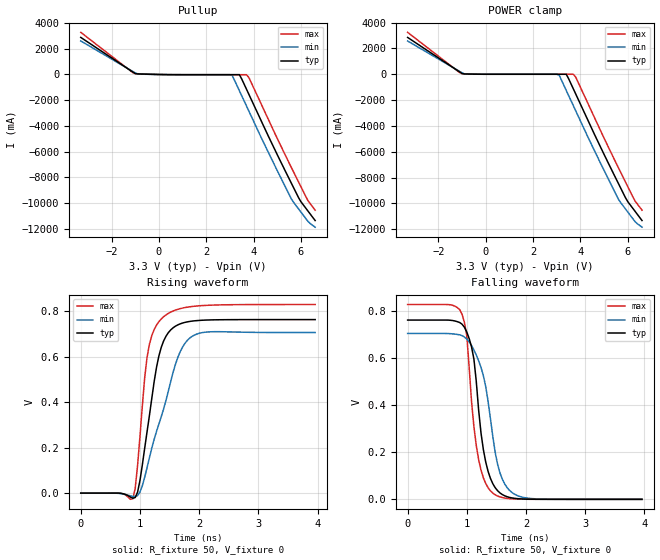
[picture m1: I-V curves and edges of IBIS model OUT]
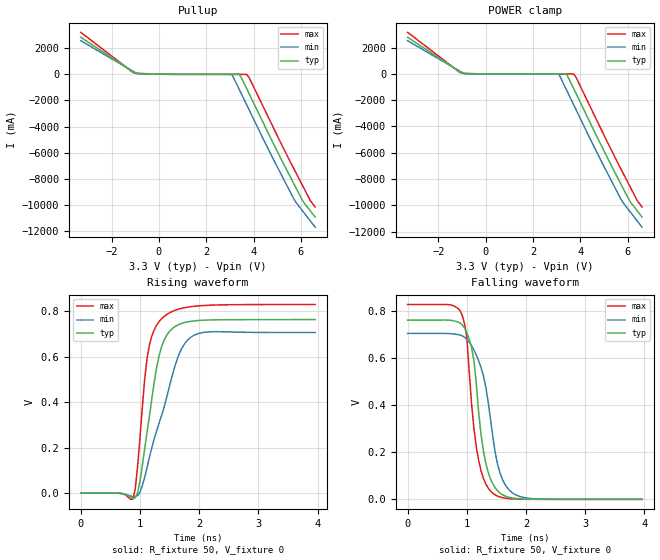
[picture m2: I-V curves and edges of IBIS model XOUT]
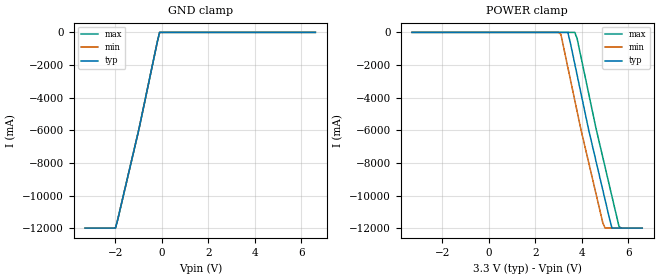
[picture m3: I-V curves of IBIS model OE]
|   IBIS File sg3225hbn_33v.ibs
[IBIS Ver]   3.2
[File name]   sg3225hbn_33v.ibs
[File Rev]   1.0
[Date]   April 7, 2016
[Source]
[Disclaimer]
Seiko Epson Corporation makes no warranty with respect to the information
contained herein.
[Copyright]
Copyright(C) 2013, Seiko Epson Corporation. All rights reserved.
|   Component SG3225HBN 3.3V
[Component]   sg3225hbn_33v
[Manufacturer]   Seiko Epson Corporation
[Package]
R_pkg   0.048   NA   NA
L_pkg   0.48n   NA   NA
C_pkg   0.21p   NA   NA
[Pin] signal_name   model_name   R_pin   L_pin   C_pin
1   OE   OE
2   NC   NC
3   GND   GND
4   OUT   OUT   0.048   0.48n   0.21p
5   XOUT   XOUT   0.048   0.48n   0.21p
6   VCC   POWER
[Diff Pin] inv_pin vdiff   tdelay_typ
4   5   0   0
| Models and submodels in the file (3): OUT (Open_source), XOUT (Open_source), OE (Input)
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[Model]   OUT
Model_type Open_source
Enable Active-High
Polarity Non-Inverting
Vref=0
Vmeas=0.375
Rref=50
Cref=0
C_comp   3.20p   2.99p   3.64p
[Temperature Range] 25   85   -40
[Voltage Range]   3.3   2.97   3.63
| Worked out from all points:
|   slope of the pullup table from 0 to 0.495 V, typ, clamps not added: 39.7 ohm
|   POWER clamp passes 1 mA (typ) near -0.15 V on its own axis
|   falling waveform, R_fixture 50, V_fixture 0: 20-80 % time 216ps typ, 293ps min, 193ps max; typ from 0.763 V to 0 V
|   rising waveform, R_fixture 50, V_fixture 0: 20-80 % time 272ps typ, 451ps min, 195ps max; typ from 0 V to 0.763 V
[Pullup]
-3.3V     2.881A     2.607A     3.275A
-1V       78.43mA    123.5mA    70.06mA
-500mV    22.06mA    15.05mA    31.55mA
3V        -15.31mA   -14.25mA   -16.57mA
3.1V      -15.31mA   -78.05mA   -16.61mA
3.4V      -15.31mA   -1.262A    -16.66mA
3.7V      -1.144A    -2.447A    -16.68mA
3.8V      -1.539A    -2.842A    -236.3mA
5.6V      -8.462A    -9.681A    -7.243A
6V        -9.884A    -10.69A    -8.721A
6.3V      -10.61A    -11.42A    -9.812A
6.6V      -11.34A    -11.86A    -10.54A
[POWER Clamp]
-3.3V     2.853A     2.578A     3.249A
-1V       61.1mA     110.8mA    46.56mA
-700mV    15.18mA    8.186mA    27.06mA
3V        -158.7pA   -183.6pA   -141pA
3.1V      -166.7pA   -69.76mA   -149pA
3.4V      -190.7pA   -1.254A    -173pA
3.7V      -1.136A    -2.439A    -197pA
3.8V      -1.531A    -2.834A    -227.1mA
5.6V      -8.453A    -9.673A    -7.234A
6V        -9.874A    -10.68A    -8.712A
6.3V      -10.6A     -11.41A    -9.801A
6.6V      -11.33A    -11.84A    -10.53A
[Falling Waveform]
R_fixture=50
V_fixture=0
V_fixture_min=0
V_fixture_max=0
0s        763.3mV    706.4mV    829.6mV
920ps     745.7mV    697mV      787.6mV
1ns       712.2mV    682.3mV    696.5mV
1.08ns    649.1mV    654.8mV    415.8mV
1.2ns     379.3mV    589.9mV    169mV
1.32ns    158.2mV    478.9mV    67.16mV
1.44ns    66.19mV    266mV      26.37mV
1.6ns     20.28mV    85.77mV    7.546mV
1.84ns    3.312mV    17.45mV    1.174mV
3.96ns    0V         0V         0V
[Rising Waveform]
R_fixture=50
V_fixture=0
V_fixture_min=0
V_fixture_max=0
0s        0V         1.468uV    0V
880ps     -22.25mV   -14.76mV   -25mV
960ps     4.283mV    -10.74mV   121.6mV
1.08ns    197.1mV    69.39mV    507.5mV
1.12ns    269.5mV    111.9mV    596.9mV
1.28ns    553.2mV    271.5mV    738.8mV
1.4ns     669.2mV    370.3mV    775.8mV
1.68ns    744.4mV    622.1mV    811.3mV
1.92ns    757.7mV    695mV      821.9mV
3.96ns    763.3mV    706.3mV    829.6mV
[Ramp]
R_load=50
dV/dt_r   4.580E-1/2.704E-10   4.238E-1/4.510E-10   4.978E-1/1.934E-10
dV/dt_f   4.580E-1/2.127E-10   4.238E-1/2.913E-10   4.978E-1/1.879E-10
|[End   OUT
[Model]   XOUT
Model_type Open_source
Enable Active-High
Polarity Inverting
Vref=0
Vmeas=0.375
Rref=50
Cref=0
C_comp   3.20p   2.99p   3.64p
[Temperature Range] 25   85   -40
[Voltage Range]   3.3   2.97   3.63
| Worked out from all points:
|   slope of the pullup table from 0 to 0.495 V, typ, clamps not added: 39.7 ohm
|   POWER clamp passes 1 mA (typ) near -0.15 V on its own axis
|   falling waveform, R_fixture 50, V_fixture 0: 20-80 % time 216ps typ, 293ps min, 192ps max; typ from 0.763 V to 0 V
|   rising waveform, R_fixture 50, V_fixture 0: 20-80 % time 273ps typ, 452ps min, 197ps max; typ from 0 V to 0.763 V
[Pullup]
-3.3V     2.816A     2.555A     3.19A
-1V       77.27mA    121mA      69.81mA
-700mV    32.22mA    22.26mA    45.41mA
3.1V      -15.31mA   -73.56mA   -16.61mA
3.4V      -15.31mA   -1.191A    -16.66mA
3.7V      -1.08A     -2.31A     -16.68mA
3.8V      -1.453A    -2.683A    -222.4mA
4.7V      -4.806A    -5.998A    -3.579A
5.7V      -8.368A    -9.524A    -7.213A
6.1V      -9.742A    -10.51A    -8.614A
6.4V      -10.44A    -11.21A    -9.663A
6.6V      -10.91A    -11.68A    -10.14A
[POWER Clamp]
-3.3V     2.789A     2.526A     3.165A
-1V       60.1mA     108.6mA    46.38mA
-800mV    18.78mA    11.85mA    32.09mA
3.1V      -166.7pA   -66.07mA   -149pA
3.4V      -190.7pA   -1.184A    -173pA
3.7V      -1.072A    -2.303A    -197pA
3.8V      -1.445A    -2.676A    -214.5mA
4.7V      -4.798A    -5.991A    -3.571A
5.7V      -8.361A    -9.516A    -7.205A
6.1V      -9.734A    -10.5A     -8.606A
6.4V      -10.43A    -11.2A     -9.654A
6.6V      -10.9A     -11.67A    -10.13A
[Falling Waveform]
R_fixture=50
V_fixture=0
V_fixture_min=0
V_fixture_max=0
0s        763.3mV    706.4mV    829.6mV
920ps     744.3mV    696.5mV    785.5mV
1ns       710.4mV    681.8mV    691mV
1.08ns    646.7mV    654.5mV    406.6mV
1.2ns     370.9mV    590mV      165.3mV
1.32ns    155.2mV    478.7mV    65.67mV
1.44ns    64.98mV    265.6mV    25.78mV
1.6ns     19.89mV    85.9mV     7.377mV
1.84ns    3.241mV    17.51mV    1.149mV
3.96ns    0V         0V         0V
[Rising Waveform]
R_fixture=50
V_fixture=0
V_fixture_min=0
V_fixture_max=0
0s        0V         1.183uV    0V
880ps     -22.39mV   -14.95mV   -26.37mV
960ps     2.08mV     -10.93mV   116.5mV
1.08ns    194.8mV    70.06mV    502mV
1.12ns    267.4mV    112.9mV    592.6mV
1.28ns    549.9mV    272.8mV    737.5mV
1.4ns     667.5mV    371mV      775.1mV
1.68ns    744.1mV    622.2mV    811.1mV
1.92ns    757.6mV    695mV      821.8mV
3.96ns    763.3mV    706.3mV    829.6mV
[Ramp]
R_load=50
dV/dt_r   4.580E-1/2.716E-10   4.238E-1/4.519E-10   4.978E-1/1.946E-10
dV/dt_f   4.580E-1/2.127E-10   4.238E-1/2.912E-10   4.978E-1/1.880E-10
|[End   XOUT
[Model]   OE
Model_type Input
Vinh=2.31
Vinl=0.99
C_comp   3p   3p   3p
[Temperature Range] 25   85   -40
[Voltage Range]   3.3   2.97   3.63
[POWER Clamp Reference]3.3   2.97   3.63
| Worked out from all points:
|   GND clamp passes 1 mA (typ) near -0.10 V on its own axis
[GND Clamp]
-3.3V     -12A       -12A       -12A
-2V       -12A       -12A       -12A
-1.9V     -11.47A    -11.47A    -11.47A
-1V       -6A        -6A        -6A
-200mV    -592.5mA   -592.5mA   -592.5mA
-100mV    -33.15uA   -29.16uA   -40.33uA
6.6V      32.19uA    34.53uA    32.12uA
[POWER Clamp]
-3.3V     32.19uA    31.39uA    35.69uA
3V        -29.25uA   -28.49uA   -32.44uA
3.1V      -30.22uA   -118.5mA   -33.52uA
3.4V      -33.15uA   -2.15A     -36.76uA
3.7V      -1.947A    -4.181A    -40uA
3.8V      -2.624A    -4.859A    -389.4mA
4.3V      -6A        -8.004A    -3.775A
4.9V      -9.645A    -11.65A    -7.64A
5V        -10.25A    -12A       -8.248A
5.3V      -12A       -12A       -10.07A
5.6V      -12A       -12A       -11.89A
6.6V      -12A       -12A       -12A
